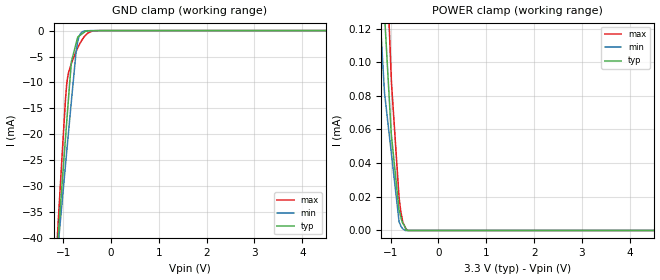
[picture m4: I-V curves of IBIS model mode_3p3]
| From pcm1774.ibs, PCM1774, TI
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|   mode_3p3 Model
[Model]   mode_3p3
Model_type   Input
Vinl = 0.99
Vinh = 2.31
|   typ   min   max
|   (nom PVT)   (fast PVT)   (slow PVT)
C_comp   8.663e-13   8.474e-13   8.760e-13
| Where nom  PVT is Nominal Process, 3.3V, 26C
|   Fast PVT is Strong Process,  3.6V, -40C
|   Slow PVT is Weak Process,   3V, 86C
[Model Spec]
|Subparameter   typ   min   max
Vinh   2.31   2.1   2.52
Vinl   0.99   0.9   1.08
[Voltage Range]   3.3   3   3.6
|Ambient Temperature   25   85   -40
|Junction Temperature
[Temperature Range]   26   86   -40
[Power Clamp Reference]   3.3   3   3.6
[GND Clamp Reference]   0   0   0
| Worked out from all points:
|   GND clamp passes 1 mA (typ) near -0.66 V on its own axis
|   POWER clamp passes 1 mA (typ) near -2.55 V on its own axis
[GND Clamp]
|   Voltage   I(typ)   I(min)   I(max)
-3.3V     -316.9mA   -268mA     -391.9mA
-1.115V   -41.24mA   -42.61mA   -38.94mA
-1.021V   -29.54mA   -33.14mA   -24.12mA
-949.2mV  -20.65mA   -25.85mA   -13.18mA
-906mV    -15.4mA    -21.5mA    -9.078mA
-825mV    -5.93mA    -13.45mA   -6.269mA
-720mV    -2.192mA   -3.574mA   -3.903mA
-648mV    -925.5uA   -754uA     -2.494mA
-567mV    -374.8uA   -93.3uA    -1.299mA
-391.2mV  -39.68uA   -226nA     -71.44uA
-243.6mV  -19.86uA   -140.7nA   -137nA
6.6V      0A         0A         0A
[POWER Clamp]
|   Voltage   I(typ)   I(min)   I(max)
-3.3V     1.567mA    1.112mA    2.083mA
-1.947V   665.3uA    484.5uA    904.5uA
-1.178V   153.2uA    106.7uA    225.9uA
-1.128V   129uA      82.03uA    191.1uA
-986.7mV  57.5uA     46.51uA    91.37uA
-981.6mV  56.08uA    45.22uA    87.77uA
-825mV    12.55uA    5.851uA    20.3uA
-787.2mV  8.182uA    2.805uA    11.29uA
-744mV    4.239uA    980.1nA    4.964uA
-693mV    1.903uA    0A         1.719uA
-653.4mV  0A         0A         377.6nA
6.6V      0A         0A         0A
